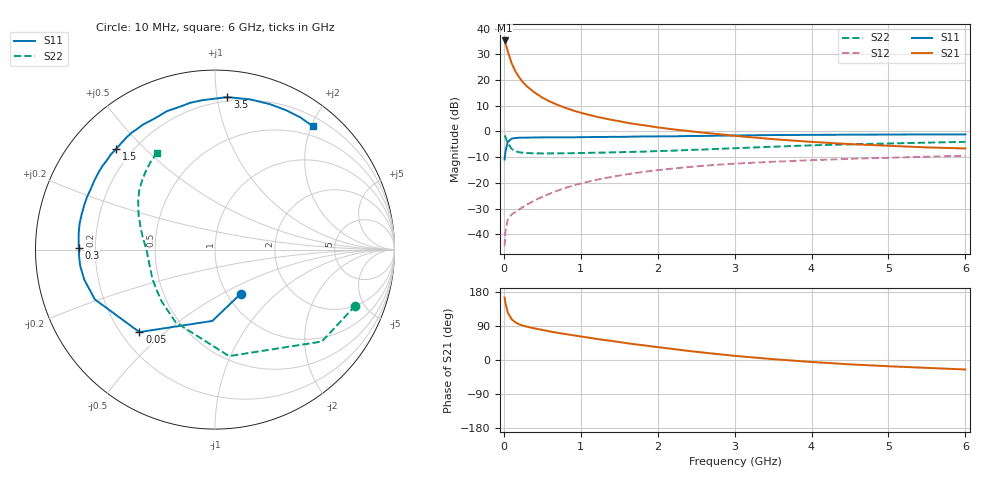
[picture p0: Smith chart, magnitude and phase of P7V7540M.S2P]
! SIEMENS Small Signal Semiconductors
! BFP196
! Si NPN RF Bipolar Junction Transistor in SOT143
! VCE = 0.75 V  IC = 40 mA
! Common Emitter S-Parameters:  May  1996
# GHz  S  MA  R  50
!  f  S11  S21  S12  S22
! GHz  MAG  ANG  MAG  ANG  MAG  ANG  MAG  ANG
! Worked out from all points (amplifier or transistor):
!   36 points, 10 MHz to 6 GHz, reference 50 ohm
!   highest |S21| = 35.4 dB at 10 MHz (marker M1)
!   |S21| within 3 dB of that: start of sweep to 39.58 MHz
!   unconditionally stable (mu >= 1): 405.7 MHz to end of sweep
!   at 250 MHz: K = 0.84, MSG = 24.2 dB, |S12| = -29.3 dB
!   at 1.4 GHz: K = 1.11, MAG = 9.0 dB, |S12| = -17.6 dB
!   at 6 GHz: K = 1.03, MAG = 0.4 dB, |S12| = -9.4 dB
!   S11 on the Smith chart (normalised r, x): 10 MHz: 1.16, -0.62; 50 MHz: 0.27, -0.41; 300 MHz: 0.14, +0.01; 1.5 GHz: 0.14, +0.41; 3.5 GHz: 0.17, +1.07; 6 GHz: 0.34, +2.02
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0.01  0.2847 -59.8  58.79 165.1  0.0059 75.8  0.8424 -21.7
0.02  0.3977 -92.1  53.08 151.1  0.011 66.5  0.7854 -40.7
0.05  0.6234 -132.5  36.57 125.8  0.0192 46.9  0.5985 -82.5
0.1  0.7248 -157.5  21.43 107.7  0.0243 41.0  0.4603 -118.5
0.15  0.7476 -167.1  14.79 99.4  0.0273 43.0  0.4144 -135.9
0.2  0.7566 -173.2  11.27 94.2  0.0305 46.0  0.3944 -146.2
0.25  0.7584 -177.5  8.994 90.6  0.0342 48.9  0.3857 -153.4
0.3  0.7593 179.2  7.546 87.9  0.0379 51.5  0.381 -157.8
0.4  0.7647 173.4  5.705 83.4  0.0457 55.2  0.3754 -164.2
0.5  0.7681 169.3  4.563 79.5  0.0536 57.5  0.3746 -168.5
0.6  0.7684 165.1  3.81 75.4  0.0621 58.4  0.3744 -171.4
0.7  0.7696 161.0  3.282 71.6  0.071 59.2  0.376 -173.8
0.8  0.7709 157.7  2.875 68.5  0.08 58.8  0.3773 -175.7
1.1  0.7776 147.1  2.114 59.0  0.1059 57.0  0.3844 179.5
1.5  0.7851 134.5  1.588 47.4  0.1391 52.1  0.3952 174.5
1.7  0.7955 128.4  1.397 41.5  0.1549 49.3  0.4024 171.5
2.2  0.8042 114.6  1.1 29.0  0.1906 41.7  0.4242 165.5
2.8  0.8296 99.5  0.885 15.2  0.2267 32.7  0.4613 157.1
3.5  0.8524 85.4  0.71 2.2  0.2584 22.6  0.5058 147.8
4.5  0.8663 69.2  0.568 -11.5  0.2939 10.5  0.5627 135.9
5.5  0.8768 57.2  0.49 -20.8  0.3241 -0.2  0.6076 126.0
6  0.8768 51.7  0.468 -25.0  0.3377 -6.0  0.6288 121.0
